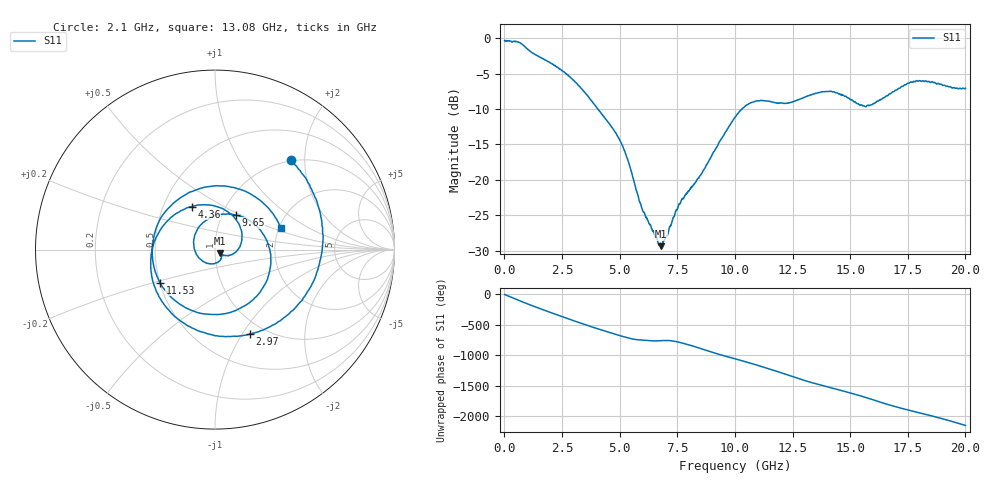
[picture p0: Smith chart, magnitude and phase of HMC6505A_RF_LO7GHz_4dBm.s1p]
! Analog Devices, Inc.
! 1 Analog Way
! Wilmington, MA 01887
! http://www.analog.com
! Date:  2021-09-17 NN
! Board Name:  EV1HMC6505ALC5 (125487-1) with HMC6505ALC5 installed
! File Description:  S-Parameters for evaluation board without connectors or board loss de-embedded
! File Generation:  Calibrated Network Analyzer
! Chip Part Number:  HMC6505A
! Chip Description:  GaAs, MMIC, IQ Upconverter
! Chip Frequency:  5.5 to 8.6 GHz
! Chip Package:  LCC, 4.9 x 4.9 x 1 mm
! Chip State:
!  Temperature:  25C
!  LO Frequency:  7GHz
!  LO Power:  4dBm
! Note:
!  Analog Devices supplies this data as a sample of measured data at the evaluation board
!  ports for this product.  Your particular data for this product may vary.
!  Analog Devices reserves the right to change this data at anytime.
!  All lines below in this file are as is from the Network Analyzer.
!Keysight Technologies,N5245A,MY49151104,A.10.65.16
!Date: Tuesday, September 14, 2021 10:46:45
!Correction: S11(Full 2 Port(1,2))
!S1P File: Measurement: S11:
# Hz S  dB  R 50
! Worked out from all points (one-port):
!   1950 points, 10 MHz to 20 GHz, reference 50 ohm
!   lowest |S11| = -29.4 dB at 6.81 GHz (marker M1), VSWR 1.07, Z = 52.7 - j2.25 ohm
!   |S11| at or under -10 dB: 4.059 GHz to 10.3 GHz (6.245 GHz wide, 87 % of centre)
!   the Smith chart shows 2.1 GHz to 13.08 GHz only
!   S11 on the Smith chart (normalised r, x): 2.1 GHz: 0.98, +1.72; 2.97 GHz: 0.86, -1.08; 4.36 GHz: 0.69, +0.36; 9.65 GHz: 1.16, +0.47; 11.53 GHz: 0.50, -0.21; 13.08 GHz: 2.06, +0.58
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1e7  -0.31 -1.6
5.6e8  -0.50 -86.3
8.4e8  -1.05 -130.9
1.08e9  -1.75 -166.6
1.62e9  -2.80 116.6
2.1e9  -3.65 49.7
2.51e9  -4.61 -6.0
2.97e9  -5.88 -67.4
3.63e9  -8.20 -152.9
4.36e9  -11.29 118.6
5.01e9  -14.41 43.1
6.81e9  -29.37 -38.8
7.51e9  -24.10 -59.8
8.81e9  -17.67 154.3
9.65e9  -12.98 59.1
1.001e10  -11.14 21.4
1.091e10  -8.86 -76.8
1.153e10  -8.92 -149.1
1.251e10  -8.97 87.0
1.308e10  -8.24 18.0
1.419e10  -7.51 -97.1
1.501e10  -8.64 179.9
1.582e10  -9.52 89.8
1.652e10  -8.27 2.4
1.751e10  -6.35 -99.7
1.849e10  -6.24 166.4
1.925e10  -6.81 89.8
2e10  -7.06 5.3
